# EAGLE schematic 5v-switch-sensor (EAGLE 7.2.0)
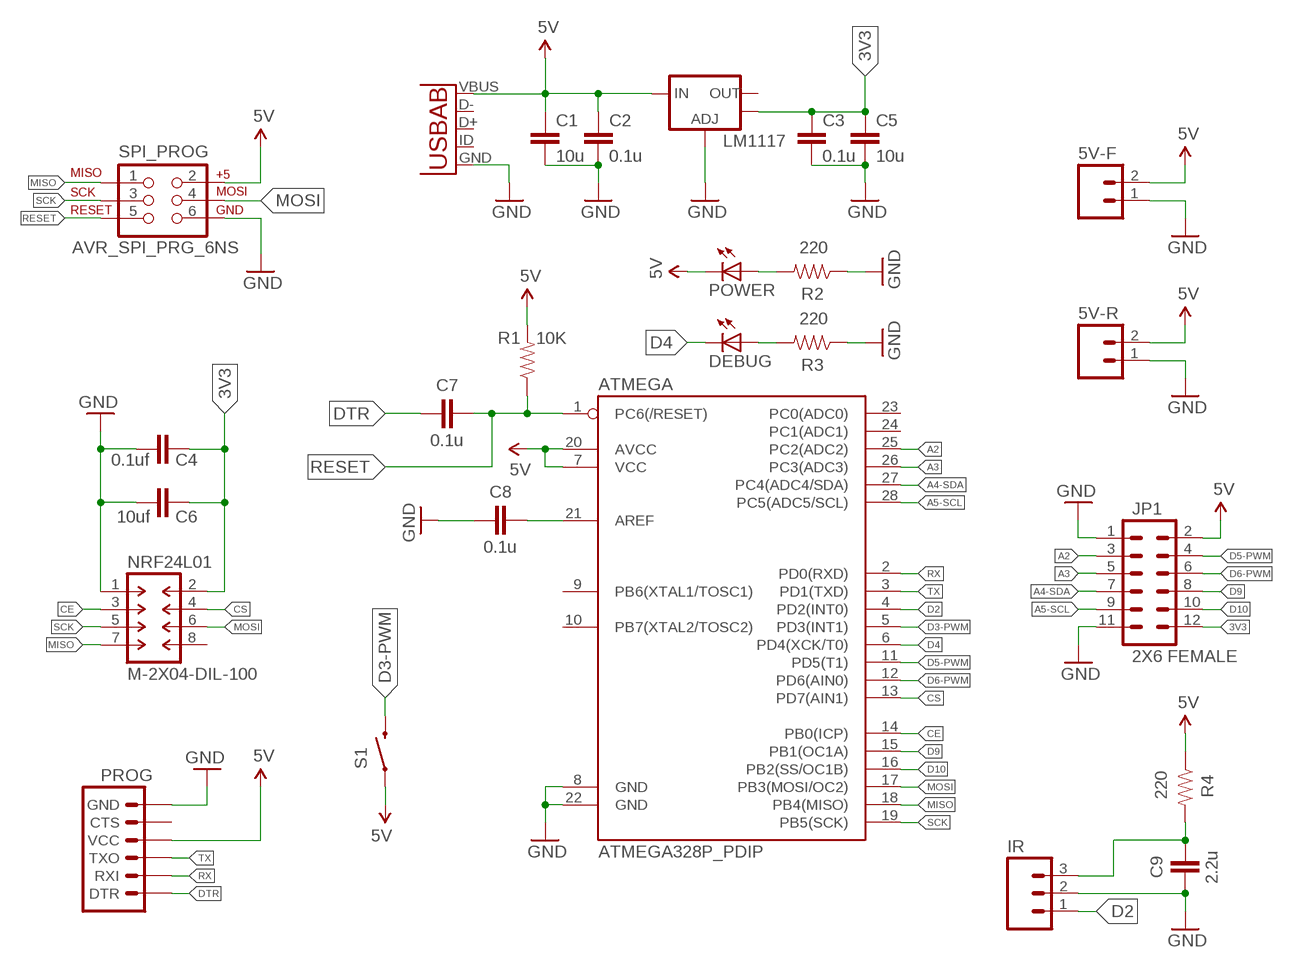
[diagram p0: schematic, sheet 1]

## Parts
5V-F  M02PTH  [1X02]
5V-R  M02PTH  [1X02]
ATMEGA  ATMEGA328P_PDIP  [DIL28-3]
C1  10u  CAP0805  [0805]
C2  0.1u  CAP0805  [0805]
C3  0.1u  CAP0805  [0805]
C4  0.1uf  CAP0805  [0805]
C5  10u  CAP0805  [0805]
C6  10uf  CAP0805  [0805]
C7  0.1u  CAP0805  [0805]
C8  0.1u  CAP0805  [0805]
C9  2.2u  CAP0805  [0805]
DEBUG  LEDCHIPLED_0805  [CHIPLED_0805]
IR  M03PTH  [1X03]
JP1  2X6 FEMALE  M06X2PTH_FEMALE  [2X6]
LM1117  V_REG_LM1117SOT223  [SOT223]
NRF24L01  M-2X04-DIL-100  [DIL-100-2X04]
POWER  LEDCHIPLED_0805  [CHIPLED_0805]
PROG  ARDUINO_SERIAL_PROGRAMPTH  [1X06]
R1  10K  RESISTOR0805-RES  [0805]
R2  220  RESISTOR0805-RES  [0805]
R3  220  RESISTOR0805-RES  [0805]
R4  220  RESISTOR0805-RES  [0805]
S1  SWITCH-MOMENTARY-2SMD-1101NE  [TACTILE-SWITCH-1101NE]
SPI_PROG  AVR_SPI_PRG_6NS  [2X3-NS]
U1  USB-AB  [USB-AB-MICRO-SMD]

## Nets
3V3: C3.1 C4.1 C5.1 C6.1 JP1.12 LM1117.4(OUT) NRF24L01.2
5V: 5V-F.2 5V-R.2 ATMEGA.7(VCC) ATMEGA.20(AVCC) C1.1 C2.1 JP1.2 LM1117.3(IN) POWER.C PROG.4(VCC) R1.2 R4.1 S1.1 SPI_PROG.2 U1.VBUS
A2: ATMEGA.25(PC2(ADC2)) JP1.3
A3: ATMEGA.26(PC3(ADC3)) JP1.5
A4-SDA: ATMEGA.27(PC4(ADC4/SDA)) JP1.7
A5-SCL: ATMEGA.28(PC5(ADC5/SCL)) JP1.9
CE: ATMEGA.14(PB0(ICP)) NRF24L01.3
CS: ATMEGA.13(PD7(AIN1)) NRF24L01.4
D2: ATMEGA.4(PD2(INT0)) IR.1
D3-PWM: ATMEGA.5(PD3(INT1)) S1.2
D4: ATMEGA.6(PD4(XCK/T0)) DEBUG.C
D5-PWM: ATMEGA.11(PD5(T1)) JP1.4
D6-PWM: ATMEGA.12(PD6(AIN0)) JP1.6
D9: ATMEGA.15(PB1(OC1A)) JP1.8
D10: ATMEGA.16(PB2(SS/OC1B)) JP1.10
DTR: C7.1 PROG.1(DTR)
GND: 5V-F.1 5V-R.1 ATMEGA.8(GND) ATMEGA.22(GND) C1.2 C2.2 C3.2 C4.2 C5.2 C6.2 C8.1 C9.1 IR.2 JP1.1 JP1.11 LM1117.1(ADJ) NRF24L01.1 PROG.6(GND) R2.1 R3.1 SPI_PROG.6 U1.GND
MISO: ATMEGA.18(PB4(MISO)) NRF24L01.7 SPI_PROG.1
MOSI: ATMEGA.17(PB3(MOSI/OC2)) NRF24L01.6 SPI_PROG.4
N$1: C9.2 IR.3 R4.2
N$2: POWER.A R2.2
N$3: ATMEGA.21(AREF) C8.2
N$4: DEBUG.A R3.2
RESET: ATMEGA.1(PC6(/RESET)) C7.2 R1.1 SPI_PROG.5
RX: ATMEGA.2(PD0(RXD)) PROG.2(RXI)
SCK: ATMEGA.19(PB5(SCK)) NRF24L01.5 SPI_PROG.3
TX: ATMEGA.3(PD1(TXD)) PROG.3(TXO)
Unconnected: ATMEGA.9(PB6(XTAL1/TOSC1)) ATMEGA.10(PB7(XTAL2/TOSC2)) ATMEGA.23(PC0(ADC0)) ATMEGA.24(PC1(ADC1)) LM1117.2(OUT) NRF24L01.8 PROG.5(CTS) U1.D+ U1.D- U1.ID(USBID)

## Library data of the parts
5V-F 5V-R = SparkFun-Connectors:M02: Standard 2-pin 0.1" header. Use with
ATMEGA = SparkFun-DigitalIC:ATMEGA328P_PDIP: uC used in the Arduino 32kb flash, 1k EEPROM, 2k SRAM This is the through-hole version of this chip.
C1-C9 = SparkFun-Capacitors:CAP: Capacitor
DEBUG POWER = adafruit:LED: LED
IR = SparkFun-Connectors:M03: Header 3 Standard 3-pin 0.1" header. Use with straight break away headers (SKU : PRT-00116), right angle break away headers (PRT-00553), swiss pins (PRT-00743), machine pins (PRT-00117), and female headers (PRT-00115). Molex polarized connector foot print use with SKU : PRT-08232 with associated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
JP1 = SparkFun-Connectors:M06X2; PROD_ID: CONN-12423
LM1117 = SparkFun-PowerIC:V_REG_LM1117: Voltage Regulator LM1117 Standard adjustable voltage regulator but in SMD form. Spark Fun Electronics SKU : COM-00595; PROD_ID: VREG-08170
NRF24L01 = con-headers-jp:M-2X04-: MALE HEADER
PROG = SparkFun-Connectors:ARDUINO_SERIAL_PROGRAM: FTDI connector footprints
R1-R4 = SparkFun-Resistors:RESISTOR: Resistor
S1 = SparkFun-Electromechanical:SWITCH-MOMENTARY-2: Various NO switches- pushbuttons, reed, etc; PROD_ID: SWCH-00815
SPI_PROG = SparkFun-Connectors:AVR_SPI_PRG_6: AVR ISP 6 Pin This is the reduced ISP connector for AVR programming. Common on Arduino. This footprint will take up less PCB space and can be used with a 10-pin to 6-pin adapter such as SKU: BOB-08508 **Special note about "TEST_POINT" package. The stop mask is on the top side, so if you want your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
U1 = SparkFun-Connectors:USB-AB: This is a USB AB connector that is compatible with USB OTG. i.e. this connector can serve as a host or device

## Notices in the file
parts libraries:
SparkFun-Connectors: Licensing: Creative Commons ShareAlike 4.0 International - https://creativecommons.org/licenses/by-sa/4.0
con-headers-jp: Copyright (C) 2008, Bob Starr
